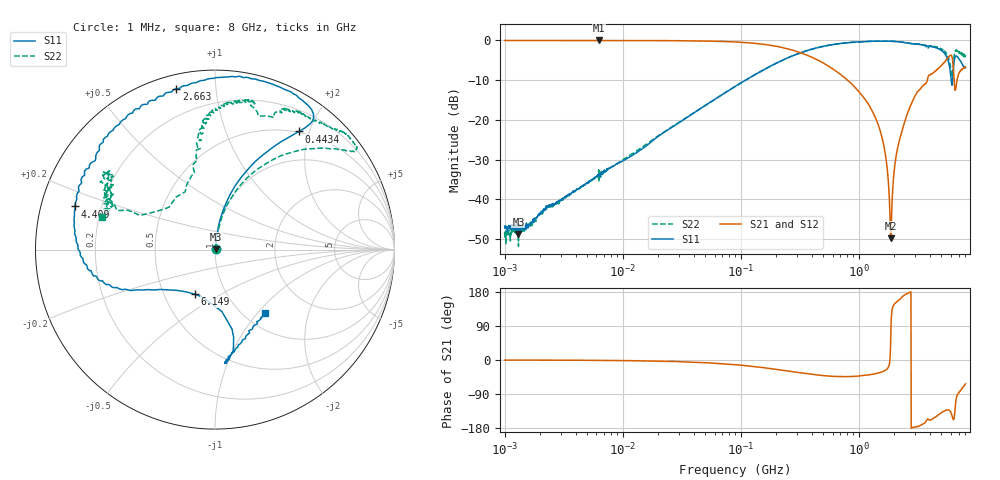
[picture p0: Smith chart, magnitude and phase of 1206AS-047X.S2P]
!s-Parameter Generated by FASTRON Sdn. Bhd.
!FASTRON P/N : 1206AS-047X
!Keysight Technologies: E5071C_MY46733604_B.14.02
!Date: Wed Nov 15 10:15:28 2023
!Version  :Rev00  Wed Nov 15 10:15:28 2023
!Data & Calibration Information:
!Freq  S11:SOLT2(ON)  S21:SOLT2(ON)  S12:SOLT2(ON)  S22:SOLT2(ON)
!PortZ  Port1:50+j0  Port2:50+j0
!When reading reference impedance value at option line is always used.
! Remarks : This data is being provided solely for informational purposes.
# Hz S dB R 50
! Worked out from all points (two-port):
!   1601 points, 1 MHz to 8 GHz, reference 50 ohm
!   highest |S21| = -0.02 dB at 6.301 MHz (marker M1); lowest = -49.8 dB at 1.869 GHz (marker M2)
!   |S21| within 3 dB of the highest: start of sweep to 314.6 MHz
!   lowest |S11| = -48.7 dB at 1.31 MHz (marker M3), VSWR 1.01, Z = 50.4 + j0.117 ohm
!   |S11| at or under -10 dB: start of sweep to 109.8 MHz; 6.067 GHz to 6.237 GHz (169.8 MHz wide, 2.76 % of centre)
!   |S22| runs from -51.7 to -0.2 dB; largest |S21 - S12| = 0.0052
!   S11 on the Smith chart (normalised r, x): 1 MHz: 1.01, +0.00; 443.4 MHz: 0.49, +1.84; 2.663 GHz: 0.07, +0.79; 4.409 GHz: 0.10, +0.15; 6.149 GHz: 0.71, -0.38; 8 GHz: 1.24, -1.10
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1000000  -46.66 10.4  -0.03 -0.3  -0.04 -0.2  -48.22 14.9
1310238  -48.67 18.4  -0.05 -0.3  -0.06 -0.2  -51.73 29.0
4479405  -36.65 72.5  -0.04 -0.7  -0.05 -0.7  -36.89 75.3
6301378  -33.89 69.2  -0.02 -1.1  -0.06 -1.0  -35.60 76.9
2.00676e7  -24.09 82.2  -0.06 -3.0  -0.08 -2.9  -23.97 81.6
8.994653e7  -11.54 76.6  -0.40 -12.4  -0.41 -12.4  -11.58 74.5
4.006501e8  -2.21 55.7  -4.25 -37.9  -4.26 -37.9  -2.22 46.5
4.433869e8  -1.86 54.6  -4.88 -39.5  -4.89 -39.5  -1.87 44.4
7.806701e8  -0.62 53.8  -9.68 -43.9  -9.69 -43.9  -0.62 36.2
1.272209e9  -0.23 63.7  -17.21 -38.2  -17.22 -38.3  -0.22 35.9
1.581568e9  -0.22 72.1  -24.67 -31.0  -24.67 -31.1  -0.20 37.9
1.709681e9  -0.22 75.6  -30.23 -25.7  -30.24 -25.9  -0.21 38.7
1.7949e9  -0.24 78.0  -37.09 -16.5  -37.11 -16.7  -0.22 39.7
1.869468e9  -0.24 80.2  -49.80 71.1  -49.89 70.9  -0.22 40.5
2.114474e9  -0.33 87.0  -27.58 154.2  -27.62 154.0  -0.32 42.2
2.662964e9  -0.71 103.5  -17.44 177.6  -17.47 177.4  -0.71 49.7
3.548043e9  -1.17 133.0  -11.18 -168.1  -11.20 -168.2  -1.25 62.9
4.408619e9  -1.78 162.8  -7.89 -151.4  -7.87 -151.6  -1.51 80.9
5.416325e9  -3.62 -164.6  -5.20 -133.1  -5.18 -133.4  -2.98 93.8
6.149367e9  -11.30 -114.6  -4.05 -145.6  -4.04 -146.0  -8.78 126.6
6.766244e9  -4.03 -85.0  -10.37 -95.3  -10.35 -95.9  -2.42 145.3
8e9  -6.91 -51.6  -6.74 -63.1  -6.77 -63.6  -3.70 164.1
